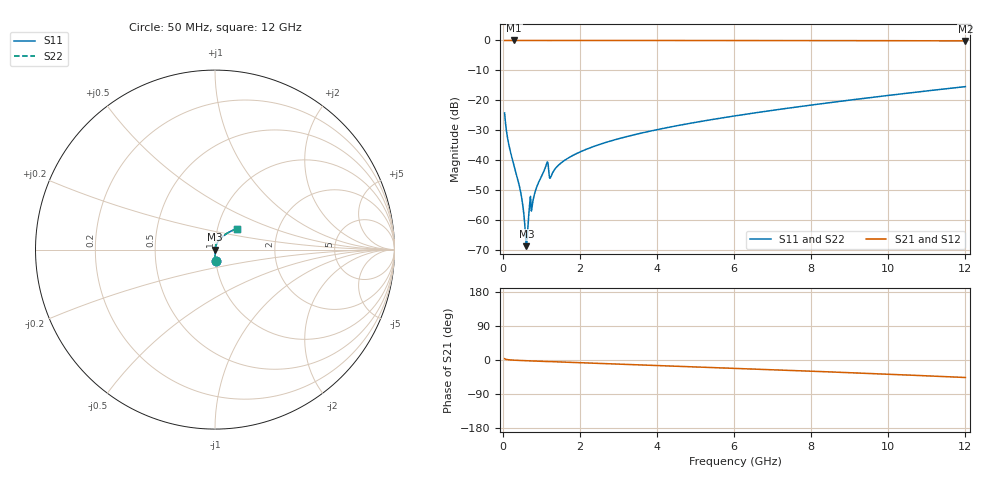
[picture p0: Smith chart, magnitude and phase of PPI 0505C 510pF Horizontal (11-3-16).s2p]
# MHz S MA R 50
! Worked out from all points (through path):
!   1601 points, 50 MHz to 12 GHz, reference 50 ohm
!   highest |S21| = 0.00 dB at 296.5 MHz (marker M1); lowest = -0.1 dB at 12 GHz (marker M2)
!   group delay of S21, straight-line fit = 10.7 ps
!   lowest |S11| = -68.6 dB at 617.6 MHz (marker M3), VSWR 1.00, Z = 50 + j0.00199 ohm
!   |S11| at or under -10 dB: start of sweep to end of sweep
!   |S22| runs from -68.6 to -15.4 dB; largest |S21 - S12| = 0
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50  0.06182 -86.5  0.9979 3.4  0.9979 3.4  0.06182 -86.5
169.5  0.01704 -88.8  0.9996 0.4  0.9996 0.4  0.01704 -88.8
296.4688  0.008157 -88.5  0.9997 -0.5  0.9997 -0.5  0.008157 -88.5
460.7812  0.003082 -85.3  0.9996 -1.3  0.9996 -1.3  0.003082 -85.3
513.0625  0.001965 -81.7  0.9996 -1.5  0.9996 -1.5  0.001965 -81.7
580.2812  0.0007347 -63.0  0.9996 -1.8  0.9996 -1.8  0.0007347 -63.0
617.625  0.0003715 3.1  0.9996 -1.9  0.9996 -1.9  0.0003715 3.1
640.0312  0.0005846 46.6  0.9996 -2.0  0.9996 -2.0  0.0005846 46.6
699.7812  0.001853 66.9  0.9993 -2.3  0.9993 -2.3  0.001853 66.9
744.5938  0.001428 49.7  0.9991 -2.4  0.9991 -2.4  0.001428 49.7
796.875  0.002304 76.0  0.9995 -2.6  0.9995 -2.6  0.002304 76.0
901.4375  0.003862 80.3  0.9995 -3.1  0.9995 -3.1  0.003862 80.3
1118.031  0.007971 75.7  0.9985 -4.0  0.9985 -4.0  0.007971 75.7
1259.938  0.005528 72.2  0.9986 -4.3  0.9986 -4.3  0.005528 72.2
1528.812  0.009223 81.2  0.9993 -5.3  0.9993 -5.3  0.009223 81.2
2044.156  0.01419 80.5  0.9992 -7.2  0.9992 -7.2  0.01419 80.5
2880.656  0.02182 78.1  0.999 -10.3  0.999 -10.3  0.02182 78.1
4038.312  0.03291 74.3  0.9985 -14.5  0.9985 -14.5  0.03291 74.3
6025  0.05525 67.2  0.9973 -21.9  0.9973 -21.9  0.05525 67.2
8019.156  0.084 59.8  0.995 -29.6  0.995 -29.6  0.084 59.8
10013.31  0.1215 51.8  0.9908 -37.6  0.9908 -37.6  0.1215 51.8
12000  0.1698 43.4  0.9834 -46.2  0.9834 -46.2  0.1698 43.4
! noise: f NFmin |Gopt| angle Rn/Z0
50  0.0002949  0.8249  0.2233  0.0003539
1372  0.003099  0.5996  4.256  0.001424
2701  0.004274  0.4742  8.137  0.001374
4031  0.005696  0.4309  11.9  0.001634
5360  0.007048  0.4034  15.51  0.001881
6682  0.008366  0.3856  18.94  0.002125
8012  0.009695  0.3746  22.21  0.002381
9341  0.01106  0.3693  25.32  0.002659
1.067e+04  0.01247  0.3688  28.29  0.002968
1.2e+04  0.01397  0.3727  31.12  0.00332
